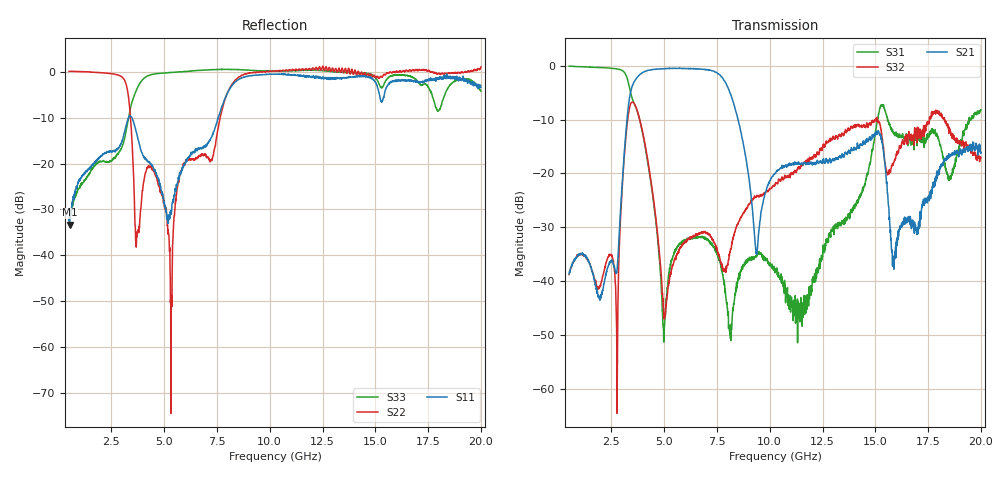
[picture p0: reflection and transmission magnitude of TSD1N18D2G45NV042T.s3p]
# MHZ S RI R 50
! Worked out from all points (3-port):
!   1951 points, 500 MHz to 20 GHz, reference 50 ohm
!   strongest paths, dB at 500 MHz, 5.37 GHz, 10.25 GHz, 15.13 GHz, 20 GHz:
!     S21: -38.7, -0.5, -20.0, -12.2, -16.1
!     S32: -38.8, -37.6, -22.1, -10.5, -17.1
!     S31: 0.0, -35.9, -37.7, -9.8, -8.2
!   lowest |S11| = -33.3 dB at 520 MHz (marker M1), VSWR 1.04, Z = 50 - j2.17 ohm
!   |S11| at or under -10 dB: start of sweep to 3.315 GHz; 3.473 GHz to 7.56 GHz (4.087 GHz wide, 74.1 % of centre)
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500  -0.00176 -0.0242  0.00436 0.0102  0.9455 -0.3088
     0.00456 0.0107  0.8567 -0.5305  0.0055 0.0102
     0.9454 -0.3081  0.00539 0.0102  -0.00568 -0.023
520  0.000895 -0.0216  0.00464 0.0107  0.9402 -0.3212
     0.005 0.0112  0.8436 -0.5496  0.00586 0.0105
     0.9404 -0.3219  0.00599 0.0103  -0.009 -0.0233
2760  -0.0716 -0.1208  -0.00296 -0.0113  -0.4911 -0.7966
      -0.00343 -0.0117  -0.8995 0.2229  0.00158 0.00121
      -0.4939 -0.7971  0.00183 0.000884  0.0691 0.1012
3500  -0.2927 -0.0841  -0.5772 -0.3181  -0.4807 0.1063
      -0.5755 -0.3201  0.1385 -0.0113  0.3946 0.2446
      -0.4782 0.107  0.3941 0.2409  -0.4806 0.0522
5330  0.00781 -0.03  0.6645 0.675  -0.00282 -0.0136
      0.6653 0.677  0.00077 -0.00202  -0.00441 -0.012
      -0.00341 -0.0151  -0.00445 -0.0115  0.4536 -0.8682
7550  0.254 -0.171  0.3228 -0.7877  -0.0135 -0.0112
      0.3155 -0.7821  0.1634 0.1732  -0.00854 0.017
      -0.0127 -0.0106  -0.0088 0.0162  -0.7203 -0.7731
9370  -0.3814 -0.8335  -0.00115 -0.0182  0.0141 -0.00744
      0.000848 -0.0179  0.0632 -0.9802  -0.049 0.0308
      0.0143 -0.00885  -0.051 0.033  -0.929 -0.4317
10250  -0.6716 -0.655  0.0846 -0.0527  0.00504 -0.0106
       0.0844 -0.053  -0.2522 -0.9752  -0.053 0.0526
       0.00547 -0.0119  -0.0558 0.0546  -0.9766 -0.2693
16210  -0.7361 -0.295  -0.0119 -0.034  0.0857 0.1889
       0.0061 -0.0323  -0.9058 0.4328  0.1138 0.1127
       0.0737 0.2087  0.1382 0.1108  -0.1207 0.9101
20000  -0.2253 0.633  -0.1232 -0.0839  0.4098 0.0782
       -0.0957 -0.1241  -1.1 -0.2352  -0.0412 -0.1424
       0.3827 0.0731  -0.0763 -0.1167  -0.2309 0.5682
